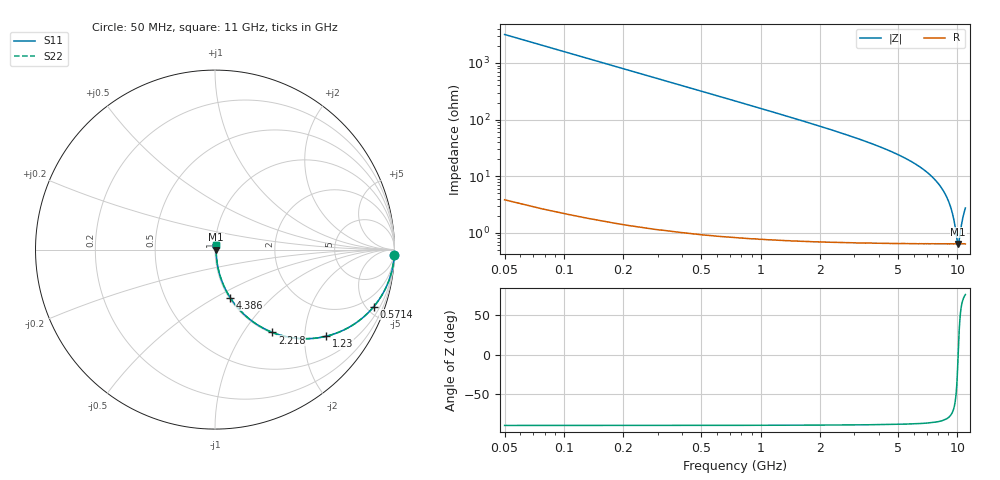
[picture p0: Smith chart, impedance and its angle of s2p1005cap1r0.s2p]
!	AVX	Thin	Film	Operation
!	Date:	March 2012
!	Description: Ultra-Miniature 01005 Size ACCU - P® Thin Film RF / Microwave Capacitor
!	Part Number:  C005YK1R0ABSTR
!	Serial	Measurements
#	MHz	S	db	R	50
!	S11	S21	S12	S22
!	dB	Phase	dB	Phase	dB	Phase	dB	Phase
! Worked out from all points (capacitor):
!   400 points, 50 MHz to 11 GHz, reference 50 ohm
!   read as one part in series: C = 1 pF near 104.9 MHz
!   lowest |Z| = 638 mohm at 10.09 GHz (marker M1)
!   series resonance near 10.11 GHz, so ESL is about 250 pH
!   S11 on the Smith chart (normalised r, x): 50 MHz: 1, -64; 571.4 MHz: 1.02, -5.55; 1.23 GHz: 1.01, -2.55; 2.218 GHz: 1.01, -1.37; 4.386 GHz: 1.01, -0.59; 11 GHz: 1.01, +0.05
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50  -0.00 -1.8  -30.06 88.1  -30.06 88.1  -0.00 -1.8
77.444  -0.01 -2.8  -26.27 87.1  -26.27 87.1  -0.01 -2.8
104.887  -0.02 -3.8  -23.64 86.1  -23.64 86.1  -0.02 -3.8
214.662  -0.08 -7.7  -17.48 82.2  -17.48 82.2  -0.08 -7.7
379.323  -0.24 -13.4  -12.69 76.4  -12.69 76.4  -0.24 -13.4
571.429  -0.54 -19.8  -9.41 70.0  -9.41 70.0  -0.54 -19.8
873.308  -1.17 -28.9  -6.32 60.9  -6.32 60.9  -1.17 -28.9
1230.075  -2.11 -38.0  -4.22 51.7  -4.22 51.7  -2.11 -38.0
1888.722  -4.04 -50.6  -2.24 38.9  -2.24 38.9  -4.04 -50.6
2218.045  -5.01 -55.3  -1.70 34.2  -1.70 34.2  -5.01 -55.3
3700  -9.19 -68.7  -0.61 20.3  -0.61 20.3  -9.19 -68.7
4386.09  -11.03 -72.4  -0.41 16.3  -0.41 16.3  -11.03 -72.4
5538.722  -14.16 -76.9  -0.23 11.3  -0.23 11.3  -14.16 -76.9
7350  -19.91 -80.6  -0.10 5.8  -0.10 5.8  -19.91 -80.6
8420.301  -24.78 -80.4  -0.07 3.3  -0.07 3.3  -24.78 -80.4
9188.722  -30.32 -76.3  -0.06 1.7  -0.06 1.7  -30.32 -76.3
9600.376  -35.24 -67.5  -0.06 0.9  -0.06 0.9  -35.24 -67.5
10012.03  -43.10 -24.6  -0.06 0.2  -0.06 0.2  -43.10 -24.6
10094.36  -43.92 -3.3  -0.06 0.0  -0.06 0.0  -43.92 -3.3
10204.14  -43.06 25.2  -0.06 -0.2  -0.06 -0.2  -43.06 25.2
10615.79  -35.57 66.7  -0.06 -0.9  -0.06 -0.9  -35.57 66.7
11000  -31.28 75.0  -0.06 -1.5  -0.06 -1.5  -31.28 75.0
